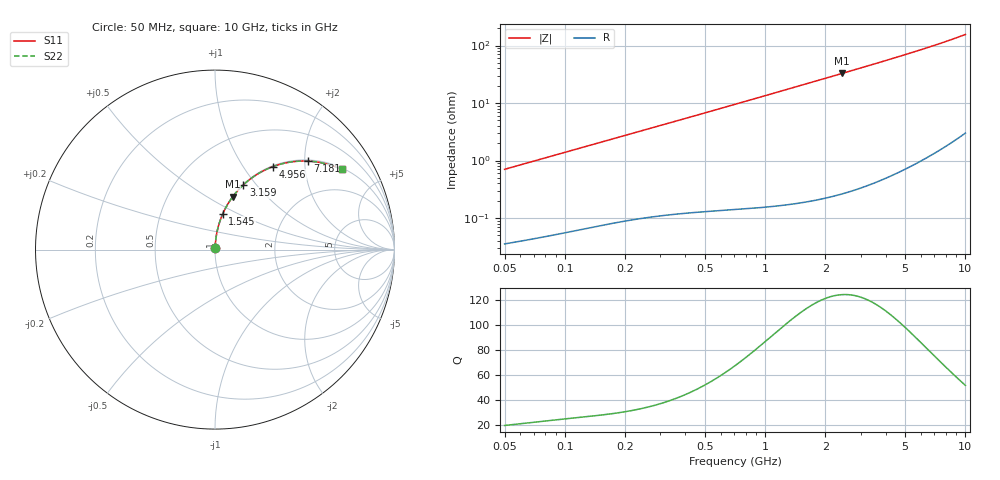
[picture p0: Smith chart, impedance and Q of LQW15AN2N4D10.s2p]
!Murata Part Number: LQW15AN2N4D10
!These Parameters are Measured in Series Mode Connection
!  o--[Z]--o
!Port1  Port2
!  o-------o
!Freq. Start=50[MHz] Stop=10[GHz], 401[Steps]
# Hz S RI R 50
!Freq.(Hz)	S 11(Real)	S 11(Imag)	S 21(Real)	S 21(Imag)	S 12(Real)	S 12(Imag)	S 22(Real)	S 22(Imag)
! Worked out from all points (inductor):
!   401 points, 50 MHz to 10 GHz, reference 50 ohm
!   read as one part in series: L = 2.23 nH near 51.34 MHz
!   highest Q = 124 at 2.424 GHz (marker M1), where L = 2.15 nH
!   S11 on the Smith chart (normalised r, x): 50 MHz: 1.00, +0.01; 1.545 GHz: 1.00, +0.42; 3.159 GHz: 1.01, +0.86; 4.956 GHz: 1.01, +1.38; 7.181 GHz: 1.03, +2.08; 10 GHz: 1.06, +3.12
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5e7  0.000405 0.00704  0.9996 -0.00704  0.9996 -0.00704  0.000405 0.00704
5.134228e7  0.000413 0.00722  0.9996 -0.00722  0.9996 -0.00722  0.000413 0.00722
1.214486e8  0.000917 0.0168  0.9991 -0.0168  0.9991 -0.0168  0.000917 0.0168
1.956524e8  0.00159 0.0267  0.9984 -0.0267  0.9984 -0.0267  0.00159 0.0267
2.949953e8  0.00268 0.0399  0.9973 -0.0399  0.9973 -0.0399  0.00268 0.0399
4.689809e8  0.00524 0.0629  0.9948 -0.0629  0.9948 -0.0629  0.00524 0.0629
7.071068e8  0.0103 0.094  0.9897 -0.094  0.9897 -0.094  0.0103 0.094
1.066141e9  0.0216 0.14  0.9784 -0.14  0.9784 -0.14  0.0216 0.14
1.544852e9  0.0431 0.1986  0.9569 -0.1986  0.9569 -0.1986  0.0431 0.1986
1.717543e9  0.0525 0.2188  0.9475 -0.2188  0.9475 -0.2188  0.0525 0.2188
2.067491e9  0.074 0.2577  0.926 -0.2577  0.926 -0.2577  0.074 0.2577
2.423676e9  0.0989 0.2945  0.9011 -0.2945  0.9011 -0.2945  0.0989 0.2945
2.766943e9  0.1253 0.3271  0.8747 -0.3271  0.8747 -0.3271  0.1253 0.3271
3.158828e9  0.1579 0.3605  0.8421 -0.3605  0.8421 -0.3605  0.1579 0.3605
3.654301e9  0.2017 0.3969  0.7983 -0.3969  0.7983 -0.3969  0.2017 0.3969
4.171863e9  0.2494 0.4281  0.7506 -0.4281  0.7506 -0.4281  0.2494 0.4281
4.955797e9  0.3231 0.4626  0.6769 -0.4626  0.6769 -0.4626  0.3231 0.4626
6.045081e9  0.4228 0.4882  0.5772 -0.4882  0.5772 -0.4882  0.4228 0.4882
7.181012e9  0.5184 0.4929  0.4816 -0.4929  0.4816 -0.4929  0.5184 0.4929
8.418147e9  0.6094 0.48  0.3906 -0.48  0.3906 -0.48  0.6094 0.48
9.738562e9  0.6908 0.4529  0.3092 -0.4529  0.3092 -0.4529  0.6908 0.4529
1e10  0.7051 0.4465  0.2949 -0.4465  0.2949 -0.4465  0.7051 0.4465
